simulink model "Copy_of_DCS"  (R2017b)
settings: Solver=FixedStepDiscrete  StartTime=0.0  StopTime=10.0  FixedStep=0.01  RelTol=1e-3  EnableMultiTasking=on
undefined symbols (not defined in the file): ASWTYPE_FALSE, CaDCS_2569BattFctyName_numb, CaDCS_2576SoftVer_numb, CcDCS_2567BattCap_Ah, CcDCS_2568BattVolt_V, CcDCS_2570BattSer_numb, CcDCS_2571BattPrdctDay_D, CcDCS_2571BattPrdctMon_M, CcDCS_2571BattPrdctYr_Y, CcDCS_2572BattChrgCt_numb, CcDCS_2574Resv_numb, CcDCS_2816MaxCellVoltPermit_V, CcDCS_2817MaxCurPermit_A, CcDCS_2818RateEgy_Kwh, CcDCS_2819MaxVoltPermit_V, CcDCS_2820MaxTempPermit_C, CcDCS_3072ChrgVoltReqAdd_V, CcDCS_CMUQnty_numb, CeDCS_2566BattType_enum, CeDCS_2573BattPrpty_enum, CeDCS_3074ChrgMode_enum, CeDCS_FltLevel_enum, DCS_2565Ver_NUMB, DCS_BROAA_NUMB, DCS_CONSTF1_NUMB, DCS_ONE_NUMB, DCS_THOUSAND_NUMB, DCS_ZERO_NUMB, Enum_CTCCtrCtlConnMode, Enum_CTCCtrCtlState, Enum_ISOHVIsoFltLevel, Enum_LDPDCChrgPlugTempState, Enum_SOPChrgPwrState
libraries: AIWAYS_Powertrain_BMS_lib x75
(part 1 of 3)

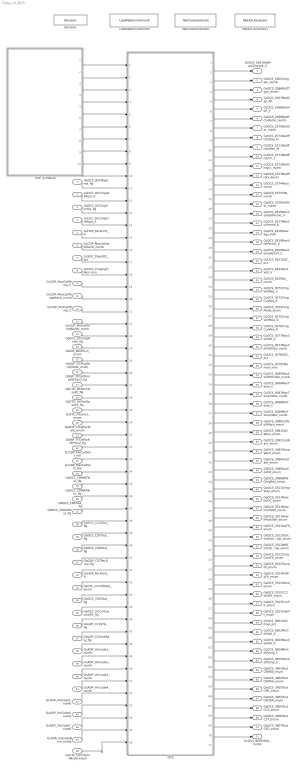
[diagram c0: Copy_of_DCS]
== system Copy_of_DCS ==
  GbDCC_BSTMsgCmd_flg : Inport
  GcDCC_DCChrgVoltRqst_V : Inport  Port=2
  GbDCC_DCChrgVerSta_flg : Inport  Port=3
  GcDCC_DCChrgCrntRqst_A : Inport  Port=4
  GcHDP_PackCrnt_A : Inport  Port=5
  GcCDP_MaxCellVoltNumb_numb : Inport  Port=6
  GcSOC_DispSOC_pct : Inport  Port=7
  GcDCC_ChrgingTiRem_min : Inport  Port=8
  GcCDP_MaxCellTemp_C : Inport  Port=9
  GcCDP_MaxCellTempNumb_numb : Inport  Port=10
  GcCDP_MinCellTemp_C : Inport  Port=11
  GcCDP_MinCellTempNumb_numb : Inport  Port=12
  GbDCC_DCChrgFinish_flg : Inport  Port=13
  GeISO_ResFltLvl_enum : Inport  Port=14
  GeLDP_DCPlugTempState_enum : Inport  Port=15
  GbISP_TFCellTempHiFltLv2_flg : Inport  Port=16
  GbCTD_DCPosCloseFlt_flg : Inport  Port=17
  GbCTD_DCPosOpenFlt_flg : Inport  Port=18
  GeFTC_FltLevel_enum : Inport  Port=19
  GeSOP_ChrgPwrState_enum : Inport  Port=20
  GbISP_TFCellVoltHiFltLv2_flg : Inport  Port=21
  GcCDP_MinCellVolt_mV : Inport  Port=22
  GcCDP_MaxCellVolt_mV : Inport  Port=23
  GbDCC_CRM00Tout_flg : Inport  Port=24
  GbDCC_CRMAATout_flg : Inport  Port=25
  GbDCC_CMLTout_flg : Inport  Port=26
  GbDCC_CROAATout_flg : Inport  Port=27
  GbDCC_CCSTout_flg : Inport  Port=28
  GbDCC_CSTTout_flg : Inport  Port=29
  GbDCC_CSDTout_flg : Inport  Port=30
  GbGDP_CSTRecOnce_flg : Inport  Port=31
  GcHDP_PackVolt_V : Inport  Port=32
  GeCTC_CtrCtlState_enum : Inport  Port=33
  GbDCC_CROTout_flg : Inport  Port=34
  GbDCC_DCCrntUnctrolFlt_flg : Inport  Port=35
  GbLDP_CC2STG_flg : Inport  Port=36
  GbLDP_CC2VoltRaty_flg : Inport  Port=37
  GcADP_VinCode1_numb : Inport  Port=38
  GcADP_VinCode2_numb : Inport  Port=39
  GcADP_VinCode3_numb : Inport  Port=40
  GcADP_VinCode4_numb : Inport  Port=41
  GcADP_VinCode5_numb : Inport  Port=42
  GcADP_VinCode6_numb : Inport  Port=43
  GcADP_VinCode7_numb : Inport  Port=44
  GcADP_VinCodeNum_numb : Inport  Port=45
  GeCTC_CtrCtlConnMode_enum : Inport  Port=46
  DCS : Subsystem
  GDP_Schedule : Stateflow chart  TreatAsAtomicUnit=on
  LoadMptEnvironment : AIWAYS_Powertrain_BMS_lib/Config/LoadMptEnvironment  ProjectName=Comm  SuppierID=NewPlatformUAES
  MptA2LGenerate1 : AIWAYS_Powertrain_BMS_lib/Config/MptA2LGenerate  SystemSampleTime=-1
  MptCodeGenerate1 : AIWAYS_Powertrain_BMS_lib/Config/MptCodeGenerate  SystemSampleTime=-1
  Revision : AIWAYS_Powertrain_BMS_lib/Config/Revision  curVersion='M104C104'  newVersion='M104C104'
  GcDCS_2601AlwMaxChrgVolt_V : Outport
  GcDCS_2565ChrgVer_numb : Outport  Port=2
  GeDCS_2566BattType_enum : Outport  Port=3
  GcDCS_2567BattCap_Ah : Outport  Port=4
  GcDCS_2568BattVolt_V : Outport  Port=5
  GaDCS_2569BattFctyName_numb : Outport  Port=6
  GcDCS_2570BattSer_numb : Outport  Port=7
  GcDCS_2571BattPrdctDay_D : Outport  Port=8
  GcDCS_2571BattPrdctMon_M : Outport  Port=9
  GcDCS_2571BattPrdctYr_Y : Outport  Port=10
  GcDCS_2572BattChrgCt_numb : Outport  Port=11
  GeDCS_2573BattPrpty_enum : Outport  Port=12
  GcDCS_2574Resv_numb : Outport  Port=13
  GaDCS_2575VIN_numb : Outport  Port=14
  GaDCS_2576SoftVer_numb : Outport  Port=15
  GcDCS_2816MaxCellVoltPermit_V : Outport  Port=16
  GcDCS_2817MaxCurPermit_A : Outport  Port=17
  GcDCS_2818RateEgy_Kwh : Outport  Port=18
  GcDCS_2819MaxVoltPermit_V : Outport  Port=19
  GcDCS_2820MaxTempPermit_C : Outport  Port=20
  GcDCS_2821SOC_pct : Outport  Port=21
  GcDCS_2822PackVolt_V : Outport  Port=22
  GcDCS_2829Da_numb : Outport  Port=23
  GcDCS_3072ChrgVoltReq_V : Outport  Port=24
  GcDCS_3073ChrgCurReq_A : Outport  Port=25
  GeDCS_3074ChrgMode_enum : Outport  Port=26
  GcDCS_3075ChrgVoltMea_V : Outport  Port=27
  GcDCS_3076ChrgCurMea_A : Outport  Port=28
  GcDCS_3077MaxCellVolt_V : Outport  Port=29
  GcDCS_3077MaxCellVoltGrp_numb : Outport  Port=30
  GcDCS_3078SOC_pct : Outport  Port=31
  GcDCS_3079TiRemain_min : Outport  Port=32
  GcDCS_3085MaxCellVoltIndex_numb : Outport  Port=33
  GcDCS_3086MaxTemp_C : Outport  Port=34
  GcDCS_3087MaxTempIndex_numb : Outport  Port=35
  GcDCS_3088MinTemp_C : Outport  Port=36
  GcDCS_3089MinTempIndex_numb : Outport  Port=37
  GeDCS_3090CellVoltWarn_enum : Outport  Port=38
  GeDCS_3091SOCWarn_enum : Outport  Port=39
  GeDCS_3092CurWarn_enum : Outport  Port=40
  GeDCS_3093TempWarn_enum : Outport  Port=41
  GeDCS_3094IsoState_enum : Outport  Port=42
  GeDCS_3095OutContSt_enum : Outport  Port=43
  GeDCS_3096BMSChrgRdy_enum : Outport  Port=44
  GeDCS_3511ChrgrStop_enum : Outport  Port=45
  GeDCS_3511ReachSOC_enum : Outport  Port=46
  GeDCS_3511ReachCellVolt_enum : Outport  Port=47
  GeDCS_3511ReachPackVolt_enum : Outport  Port=48
  GeDCS_3512IsoFlt_enum : Outport  Port=49
  GeDCS_3512OutContOverTemp_enum : Outport  Port=50
  GeDCS_3512BMSCompOverTemp_enum : Outport  Port=51
  GeDCS_3512ChrgContFlt_enum : Outport  Port=52
  GeDCS_3512TempFlt_enum : Outport  Port=53
  GeDCS_3512HVRlyFlt_enum : Outport  Port=54
  GeDCS_3512Other_enum : Outport  Port=55
  GeDCS_3512CC2VoltFlt_enum : Outport  Port=56
  GeDCS_3513CurrFlt_enum : Outport  Port=57
  GeDCS_3513VoltFlt_enum : Outport  Port=58
  GcDCS_3601SOCFinal_pct : Outport  Port=59
  GcDCS_3602MinCellVolt_V : Outport  Port=60
  GcDCS_3603MaxCellVolt_V : Outport  Port=61
  GcDCS_3604MinCellTemp_C : Outport  Port=62
  GcDCS_3605MaxCellTemp_C : Outport  Port=63
  GeDCS_3901ToutCRM00_enum : Outport  Port=64
  GeDCS_3902ToutCRMAA_enum : Outport  Port=65
  GeDCS_3903ToutCML_enum : Outport  Port=66
  GeDCS_3904ToutCROAA_enum : Outport  Port=67
  GeDCS_3905ToutCCS_enum : Outport  Port=68
  GeDCS_3906ToutCST_enum : Outport  Port=69
  GeDCS_3907ToutCSD_enum : Outport  Port=70
  GcDCS_BEMOther_numb : Outport  Port=71
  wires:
  DCS/1(GcDCS_2601AlwMaxChrgVolt_V) -> GcDCS_2601AlwMaxChrgVolt_V/1
  DCS/2(GcDCS_2565ChrgVer_numb) -> GcDCS_2565ChrgVer_numb/1
  DCS/3(GeDCS_2566BattType_enum) -> GeDCS_2566BattType_enum/1
  DCS/4(GcDCS_2567BattCap_Ah) -> GcDCS_2567BattCap_Ah/1
  DCS/5(GcDCS_2568BattVolt_V) -> GcDCS_2568BattVolt_V/1
  DCS/6(GaDCS_2569BattFctyName_numb) -> GaDCS_2569BattFctyName_numb/1
  DCS/7(GcDCS_2570BattSer_numb) -> GcDCS_2570BattSer_numb/1
  DCS/8(GcDCS_2571BattPrdctDay_D) -> GcDCS_2571BattPrdctDay_D/1
  DCS/9(GcDCS_2571BattPrdctMon_M) -> GcDCS_2571BattPrdctMon_M/1
  DCS/10(GcDCS_2571BattPrdctYr_Y) -> GcDCS_2571BattPrdctYr_Y/1
  DCS/11(GcDCS_2572BattChrgCt_numb) -> GcDCS_2572BattChrgCt_numb/1
  DCS/12(GeDCS_2573BattPrpty_enum) -> GeDCS_2573BattPrpty_enum/1
  DCS/13(GcDCS_2574Resv_numb) -> GcDCS_2574Resv_numb/1
  DCS/14(GaDCS_2575VIN_numb) -> GaDCS_2575VIN_numb/1
  DCS/15(GaDCS_2576SoftVer_numb) -> GaDCS_2576SoftVer_numb/1
  DCS/16(GcDCS_2816MaxCellVoltPermit_V) -> GcDCS_2816MaxCellVoltPermit_V/1
  DCS/17(GcDCS_2817MaxCurPermit_A) -> GcDCS_2817MaxCurPermit_A/1
  DCS/18(GcDCS_2818RateEgy_Kwh) -> GcDCS_2818RateEgy_Kwh/1
  DCS/19(GcDCS_2819MaxVoltPermit_V) -> GcDCS_2819MaxVoltPermit_V/1
  DCS/20(GcDCS_2820MaxTempPermit_C) -> GcDCS_2820MaxTempPermit_C/1
  DCS/21(GcDCS_2821SOC_pct) -> GcDCS_2821SOC_pct/1
  DCS/22(GcDCS_2822PackVolt_V) -> GcDCS_2822PackVolt_V/1
  DCS/23(GcDCS_2829Da_numb) -> GcDCS_2829Da_numb/1
  DCS/24(GcDCS_3072ChrgVoltReq_V) -> GcDCS_3072ChrgVoltReq_V/1
  DCS/25(GcDCS_3073ChrgCurReq_A) -> GcDCS_3073ChrgCurReq_A/1
  DCS/26(GeDCS_3074ChrgMode_enum) -> GeDCS_3074ChrgMode_enum/1
  DCS/27(GcDCS_3075ChrgVoltMea_V) -> GcDCS_3075ChrgVoltMea_V/1
  DCS/28(GcDCS_3076ChrgCurMea_A) -> GcDCS_3076ChrgCurMea_A/1
  DCS/29(GcDCS_3077MaxCellVolt_V) -> GcDCS_3077MaxCellVolt_V/1
  DCS/30(GcDCS_3077MaxCellVoltGrp_numb) -> GcDCS_3077MaxCellVoltGrp_numb/1
  DCS/31(GcDCS_3078SOC_pct) -> GcDCS_3078SOC_pct/1
  DCS/32(GcDCS_3079TiRemain_min) -> GcDCS_3079TiRemain_min/1
  DCS/33(GcDCS_3085MaxCellVoltIndex_numb) -> GcDCS_3085MaxCellVoltIndex_numb/1
  DCS/34(GcDCS_3086MaxTemp_C) -> GcDCS_3086MaxTemp_C/1
  DCS/35(GcDCS_3087MaxTempIndex_numb) -> GcDCS_3087MaxTempIndex_numb/1
  DCS/36(GcDCS_3088MinTemp_C) -> GcDCS_3088MinTemp_C/1
  DCS/37(GcDCS_3089MinTempIndex_numb) -> GcDCS_3089MinTempIndex_numb/1
  DCS/38(GeDCS_3090CellVoltWarn_enum) -> GeDCS_3090CellVoltWarn_enum/1
  DCS/39(GeDCS_3091SOCWarn_enum) -> GeDCS_3091SOCWarn_enum/1
  DCS/40(GeDCS_3092CurWarn_enum) -> GeDCS_3092CurWarn_enum/1
  DCS/41(GeDCS_3093TempWarn_enum) -> GeDCS_3093TempWarn_enum/1
  DCS/42(GeDCS_3094IsoState_enum) -> GeDCS_3094IsoState_enum/1
  DCS/43(GeDCS_3095OutContSt_enum) -> GeDCS_3095OutContSt_enum/1
  DCS/44(GeDCS_3096BMSChrgRdy_enum) -> GeDCS_3096BMSChrgRdy_enum/1
  DCS/45(GeDCS_3511ChrgrStop_enum) -> GeDCS_3511ChrgrStop_enum/1
  DCS/46(GeDCS_3511ReachSOC_enum) -> GeDCS_3511ReachSOC_enum/1
  DCS/47(GeDCS_3511ReachCellVolt_enum) -> GeDCS_3511ReachCellVolt_enum/1
  DCS/48(GeDCS_3511ReachPackVolt_enum) -> GeDCS_3511ReachPackVolt_enum/1
  DCS/49(GeDCS_3512IsoFlt_enum) -> GeDCS_3512IsoFlt_enum/1
  DCS/50(GeDCS_3512OutContOverTemp_enum) -> GeDCS_3512OutContOverTemp_enum/1
  DCS/51(GeDCS_3512BMSCompOverTemp_enum) -> GeDCS_3512BMSCompOverTemp_enum/1
  DCS/52(GeDCS_3512ChrgContFlt_enum) -> GeDCS_3512ChrgContFlt_enum/1
  DCS/53(GeDCS_3512TempFlt_enum) -> GeDCS_3512TempFlt_enum/1
  DCS/54(GeDCS_3512HVRlyFlt_enum) -> GeDCS_3512HVRlyFlt_enum/1
  DCS/55(GeDCS_3512Other_enum) -> GeDCS_3512Other_enum/1
  DCS/56(GeDCS_3512CC2VoltFlt_enum) -> GeDCS_3512CC2VoltFlt_enum/1
  DCS/57(GeDCS_3513CurrFlt_enum) -> GeDCS_3513CurrFlt_enum/1
  DCS/58(GeDCS_3513VoltFlt_enum) -> GeDCS_3513VoltFlt_enum/1
  DCS/59(GcDCS_3601SOCFinal_pct) -> GcDCS_3601SOCFinal_pct/1
  DCS/60(GcDCS_3602MinCellVolt_V) -> GcDCS_3602MinCellVolt_V/1
  DCS/61(GcDCS_3603MaxCellVolt_V) -> GcDCS_3603MaxCellVolt_V/1
  DCS/62(GcDCS_3604MinCellTemp_C) -> GcDCS_3604MinCellTemp_C/1
  DCS/63(GcDCS_3605MaxCellTemp_C) -> GcDCS_3605MaxCellTemp_C/1
  DCS/64(GeDCS_3901ToutCRM00_enum) -> GeDCS_3901ToutCRM00_enum/1
  DCS/65(GeDCS_3902ToutCRMAA_enum) -> GeDCS_3902ToutCRMAA_enum/1
  DCS/66(GeDCS_3903ToutCML_enum) -> GeDCS_3903ToutCML_enum/1
  DCS/67(GeDCS_3904ToutCROAA_enum) -> GeDCS_3904ToutCROAA_enum/1
  DCS/68(GeDCS_3905ToutCCS_enum) -> GeDCS_3905ToutCCS_enum/1
  DCS/69(GeDCS_3906ToutCST_enum) -> GeDCS_3906ToutCST_enum/1
  DCS/70(GeDCS_3907ToutCSD_enum) -> GeDCS_3907ToutCSD_enum/1
  DCS/71(GcDCS_BEMOther_numb) -> GcDCS_BEMOther_numb/1
  GDP_Schedule/1(DCS_BST_10ms()) -> DCS/1(DCS_BST_10ms)
  GDP_Schedule/2(DCS_BCL_50ms()) -> DCS/2(DCS_BCL_50ms)
  GDP_Schedule/3(DCS_BHM_250ms()) -> DCS/3(DCS_BHM_250ms)
  GDP_Schedule/4(DCS_BRM_250ms()) -> DCS/4(DCS_BRM_250ms)
  GDP_Schedule/5(DCS_BRO_250ms()) -> DCS/5(DCS_BRO_250ms)
  GDP_Schedule/6(DCS_BCS_250ms()) -> DCS/6(DCS_BCS_250ms)
  GDP_Schedule/7(DCS_BSM_250ms()) -> DCS/7(DCS_BSM_250ms)
  GDP_Schedule/8(DCS_BSD_250ms()) -> DCS/8(DCS_BSD_250ms)
  GDP_Schedule/9(DCS_BEM_250ms()) -> DCS/9(DCS_BEM_250ms)
  GDP_Schedule/10(DCS_BCP_500ms()) -> DCS/10(DCS_BCP_500ms)
  GbDCC_BSTMsgCmd_flg/1 -> DCS/11(GbDCC_BSTMsgCmd_flg)
  GcDCC_DCChrgVoltRqst_V/1 -> DCS/12(GcDCC_DCChrgVoltRqst_V)
  GbDCC_DCChrgVerSta_flg/1 -> DCS/13(GbDCC_DCChrgVerSta_flg)
  GcDCC_DCChrgCrntRqst_A/1 -> DCS/14(GcDCC_DCChrgCrntRqst_A)
  GcHDP_PackCrnt_A/1 -> DCS/15(GcHDP_PackCrnt_A)
  GcCDP_MaxCellVoltNumb_numb/1 -> DCS/16(GcCDP_MaxCellVoltNumb_numb)
  GcSOC_DispSOC_pct/1 -> DCS/17(GcSOC_DispSOC_pct)
  GcDCC_ChrgingTiRem_min/1 -> DCS/18(GcDCC_ChrgingTiRem_min)
  GcCDP_MaxCellTemp_C/1 -> DCS/19(GcCDP_MaxCellTemp_C)
  GcCDP_MaxCellTempNumb_numb/1 -> DCS/20(GcCDP_MaxCellTempNumb_numb)
  GcCDP_MinCellTemp_C/1 -> DCS/21(GcCDP_MinCellTemp_C)
  GcCDP_MinCellTempNumb_numb/1 -> DCS/22(GcCDP_MinCellTempNumb_numb)
  GbDCC_DCChrgFinish_flg/1 -> DCS/23(GbDCC_DCChrgFinish_flg)
  GeISO_ResFltLvl_enum/1 -> DCS/24(GeISO_ResFltLvl_enum)
  GeLDP_DCPlugTempState_enum/1 -> DCS/25(GeLDP_DCPlugTempState_enum)
  GbISP_TFCellTempHiFltLv2_flg/1 -> DCS/26(GbISP_TFCellTempHiFltLv2_flg)
  GbCTD_DCPosCloseFlt_flg/1 -> DCS/27(GbCTD_DCPosCloseFlt_flg)
  GbCTD_DCPosOpenFlt_flg/1 -> DCS/28(GbCTD_DCPosOpenFlt_flg)
  GeFTC_FltLevel_enum/1 -> DCS/29(GeFTC_FltLevel_enum)
  GeSOP_ChrgPwrState_enum/1 -> DCS/30(GeSOP_ChrgPwrState_enum)
  GbISP_TFCellVoltHiFltLv2_flg/1 -> DCS/31(GbISP_TFCellVoltHiFltLv2_flg)
  GcCDP_MinCellVolt_mV/1 -> DCS/32(GcCDP_MinCellVolt_mV)
  GcCDP_MaxCellVolt_mV/1 -> DCS/33(GcCDP_MaxCellVolt_mV)
  GbDCC_CRM00Tout_flg/1 -> DCS/34(GbDCC_CRM00Tout_flg)
  GbDCC_CRMAATout_flg/1 -> DCS/35(GbDCC_CRMAATout_flg)
  GbDCC_CMLTout_flg/1 -> DCS/36(GbDCC_CMLTout_flg)
  GbDCC_CROAATout_flg/1 -> DCS/37(GbDCC_CROAATout_flg)
  GbDCC_CCSTout_flg/1 -> DCS/38(GbDCC_CCSTout_flg)
  GbDCC_CSTTout_flg/1 -> DCS/39(GbDCC_CSTTout_flg)
  GbDCC_CSDTout_flg/1 -> DCS/40(GbDCC_CSDTout_flg)
  GbGDP_CSTRecOnce_flg/1 -> DCS/41(GbGDP_CSTRecOnce_flg)
  GcHDP_PackVolt_V/1 -> DCS/42(GcHDP_PackVolt_V)
  GeCTC_CtrCtlState_enum/1 -> DCS/43(GeCTC_CtrCtlState_enum)
  GbDCC_CROTout_flg/1 -> DCS/44(GbDCC_CROTout_flg)
  GbDCC_DCCrntUnctrolFlt_flg/1 -> DCS/45(GbDCC_DCCrntUnctrolFlt_flg)
  GbLDP_CC2STG_flg/1 -> DCS/46(GbLDP_CC2STG_flg)
  GbLDP_CC2VoltRaty_flg/1 -> DCS/47(GbLDP_CC2VoltRaty_flg)
  GcADP_VinCode1_numb/1 -> DCS/48(GcADP_VinCode1_numb)
  GcADP_VinCode2_numb/1 -> DCS/49(GcADP_VinCode2_numb)
  GcADP_VinCode3_numb/1 -> DCS/50(GcADP_VinCode3_numb)
  GcADP_VinCode4_numb/1 -> DCS/51(GcADP_VinCode4_numb)
  GcADP_VinCode5_numb/1 -> DCS/52(GcADP_VinCode5_numb)
  GcADP_VinCode6_numb/1 -> DCS/53(GcADP_VinCode6_numb)
  GcADP_VinCode7_numb/1 -> DCS/54(GcADP_VinCode7_numb)
  GcADP_VinCodeNum_numb/1 -> DCS/55(GcADP_VinCodeNum_numb)
  GeCTC_CtrCtlConnMode_enum/1 -> DCS/56(GeCTC_CtrCtlConnMode_enum)

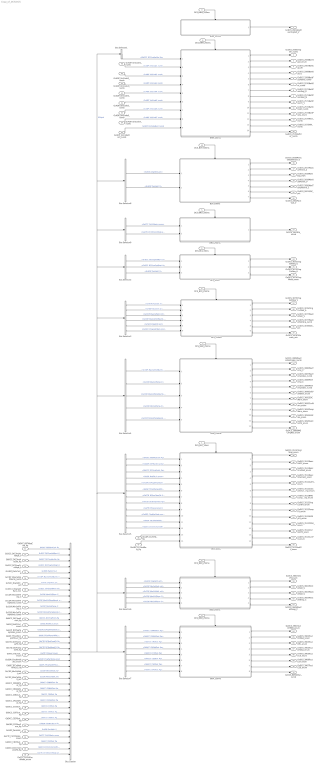
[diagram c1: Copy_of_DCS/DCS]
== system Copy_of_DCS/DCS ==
  DCS_BST_10ms : Inport
  DCS_BCL_50ms : Inport  Port=2
  DCS_BHM_250ms : Inport  Port=3
  DCS_BRM_250ms : Inport  Port=4
  DCS_BRO_250ms : Inport  Port=5
  DCS_BCS_250ms : Inport  Port=6
  DCS_BSM_250ms : Inport  Port=7
  DCS_BSD_250ms : Inport  Port=8
  DCS_BEM_250ms : Inport  Port=9
  DCS_BCP_500ms : Inport  Port=10
  GbDCC_BSTMsgCmd_flg : Inport  Port=11
  GcDCC_DCChrgVoltRqst_V : Inport  Port=12
  GbDCC_DCChrgVerSta_flg : Inport  Port=13
  GcDCC_DCChrgCrntRqst_A : Inport  Port=14
  GcHDP_PackCrnt_A : Inport  Port=15
  GcCDP_MaxCellVoltNumb_numb : Inport  Port=16
  GcSOC_DispSOC_pct : Inport  Port=17
  GcDCC_ChrgingTiRem_min : Inport  Port=18
  GcCDP_MaxCellTemp_C : Inport  Port=19
  GcCDP_MaxCellTempNumb_numb : Inport  Port=20
  GcCDP_MinCellTemp_C : Inport  Port=21
  GcCDP_MinCellTempNumb_numb : Inport  Port=22
  GbDCC_DCChrgFinish_flg : Inport  Port=23
  GeISO_ResFltLvl_enum : Inport  Port=24
  GeLDP_DCPlugTempState_enum : Inport  Port=25
  GbISP_TFCellTempHiFltLv2_flg : Inport  Port=26
  GbCTD_DCPosCloseFlt_flg : Inport  Port=27
  GbCTD_DCPosOpenFlt_flg : Inport  Port=28
  GeFTC_FltLevel_enum : Inport  Port=29
  GeSOP_ChrgPwrState_enum : Inport  Port=30
  GbISP_TFCellVoltHiFltLv2_flg : Inport  Port=31
  GcCDP_MinCellVolt_mV : Inport  Port=32
  GcCDP_MaxCellVolt_mV : Inport  Port=33
  GbDCC_CRM00Tout_flg : Inport  Port=34
  GbDCC_CRMAATout_flg : Inport  Port=35
  GbDCC_CMLTout_flg : Inport  Port=36
  GbDCC_CROAATout_flg : Inport  Port=37
  GbDCC_CCSTout_flg : Inport  Port=38
  GbDCC_CSTTout_flg : Inport  Port=39
  GbDCC_CSDTout_flg : Inport  Port=40
  GbGDP_CSTRecOnce_flg : Inport  Port=41
  GcHDP_PackVolt_V : Inport  Port=42
  GeCTC_CtrCtlState_enum : Inport  Port=43
  GbDCC_CROTout_flg : Inport  Port=44
  GbDCC_DCCrntUnctrolFlt_flg : Inport  Port=45
  GbLDP_CC2STG_flg : Inport  Port=46
  GbLDP_CC2VoltRaty_flg : Inport  Port=47
  GcADP_VinCode1_numb : Inport  Port=48
  GcADP_VinCode2_numb : Inport  Port=49
  GcADP_VinCode3_numb : Inport  Port=50
  GcADP_VinCode4_numb : Inport  Port=51
  GcADP_VinCode5_numb : Inport  Port=52
  GcADP_VinCode6_numb : Inport  Port=53
  GcADP_VinCode7_numb : Inport  Port=54
  GcADP_VinCodeNum_numb : Inport  Port=55
  GeCTC_CtrCtlConnMode_enum : Inport  Port=56
  BCL_50ms : Subsystem
  BCP_500ms : Subsystem
  BCS_250ms : Subsystem
  BEM_250ms : Subsystem
  BHM_250ms : Subsystem
  BRM_250ms : Subsystem
  BRO_250ms : Subsystem
  BSD_250ms : Subsystem
  BSM_250ms : Subsystem
  BST_10ms : Subsystem
  Bus Creator : BusCreator  Inputs=36
  Bus Selector1 : BusSelector  OutputSignals=GbDCC_DCChrgVerSta_flg
  Bus Selector2 : BusSelector  OutputSignals=GcDCC_DCChrgVoltRqst_V,GcDCC_DCChrgCrntRqst_A,GcHDP_PackVolt_V
  Bus Selector3 : BusSelector  OutputSignals=GcHDP_PackVolt_V,GcHDP_PackCrnt_A,GcCDP_MaxCellVolt_mV,GcCDP_MaxCellVoltNumb_numb,GcSOC_DispSOC_pct,GcDCC_ChrgingTiRem_min
  Bus Selector4 : BusSelector  OutputSignals=GcCDP_MaxCellVoltNumb_numb,GcCDP_MaxCellTemp_C,GcCDP_MaxCellTempNumb_numb,GcCDP_MinCellTemp_C,GcCDP_MinCellTempNumb_numb
  Bus Selector5 : BusSelector  OutputSignals=GbDCC_BSTMsgCmd_flg,GbGDP_CSTRecOnce_flg,GbDCC_DCChrgFinish_flg,GeISO_ResFltLvl_enum,GeLDP_DCPlugTempState_enum,GbISP_TFCellTempHiFltLv2_flg,GbCTD_DCPosCloseFlt_flg,GbCTD_DCPosOpenFlt_flg,GeFTC_FltLevel_enum,GeSOP_ChrgPwrState_enum,GbISP_TFCellVoltHiFltLv2_flg,GbDCC_DCCrntUnctrolFlt_flg
  Bus Selector6 : BusSelector  OutputSignals=GcSOC_DispSOC_pct,GcCDP_MinCellVolt_mV,GcCDP_MaxCellVolt_mV,GcCDP_MaxCellTemp_C,GcCDP_MinCellTemp_C
  Bus Selector7 : BusSelector  OutputSignals=GbDCC_CRM00Tout_flg,GbDCC_CRMAATout_flg,GbDCC_CMLTout_flg,GbDCC_CROAATout_flg,GbDCC_CCSTout_flg,GbDCC_CSTTout_flg,GbDCC_CSDTout_flg,GbDCC_CROTout_flg
  Bus Selector8 : BusSelector  OutputSignals=GcSOC_DispSOC_pct,GcHDP_PackVolt_V
  Bus Selector9 : BusSelector  OutputSignals=GeCTC_CtrCtlState_enum,GeCTC_CtrCtlConnMode_enum
  GcDCS_2601AlwMaxChrgVolt_V : Outport
  GcDCS_2565ChrgVer_numb : Outport  Port=2
  GeDCS_2566BattType_enum : Outport  Port=3
  GcDCS_2567BattCap_Ah : Outport  Port=4
  GcDCS_2568BattVolt_V : Outport  Port=5
  GaDCS_2569BattFctyName_numb : Outport  Port=6
  GcDCS_2570BattSer_numb : Outport  Port=7
  GcDCS_2571BattPrdctDay_D : Outport  Port=8
  GcDCS_2571BattPrdctMon_M : Outport  Port=9
  GcDCS_2571BattPrdctYr_Y : Outport  Port=10
  GcDCS_2572BattChrgCt_numb : Outport  Port=11
  GeDCS_2573BattPrpty_enum : Outport  Port=12
  GcDCS_2574Resv_numb : Outport  Port=13
  GaDCS_2575VIN_numb : Outport  Port=14
  GaDCS_2576SoftVer_numb : Outport  Port=15
  GcDCS_2816MaxCellVoltPermit_V : Outport  Port=16
  GcDCS_2817MaxCurPermit_A : Outport  Port=17
  GcDCS_2818RateEgy_Kwh : Outport  Port=18
  GcDCS_2819MaxVoltPermit_V : Outport  Port=19
  GcDCS_2820MaxTempPermit_C : Outport  Port=20
  GcDCS_2821SOC_pct : Outport  Port=21
  GcDCS_2822PackVolt_V : Outport  Port=22
  GcDCS_2829Da_numb : Outport  Port=23
  GcDCS_3072ChrgVoltReq_V : Outport  Port=24
  GcDCS_3073ChrgCurReq_A : Outport  Port=25
  GeDCS_3074ChrgMode_enum : Outport  Port=26
  GcDCS_3075ChrgVoltMea_V : Outport  Port=27
  GcDCS_3076ChrgCurMea_A : Outport  Port=28
  GcDCS_3077MaxCellVolt_V : Outport  Port=29
  GcDCS_3077MaxCellVoltGrp_numb : Outport  Port=30
  GcDCS_3078SOC_pct : Outport  Port=31
  GcDCS_3079TiRemain_min : Outport  Port=32
  GcDCS_3085MaxCellVoltIndex_numb : Outport  Port=33
  GcDCS_3086MaxTemp_C : Outport  Port=34
  GcDCS_3087MaxTempIndex_numb : Outport  Port=35
  GcDCS_3088MinTemp_C : Outport  Port=36
  GcDCS_3089MinTempIndex_numb : Outport  Port=37
  GeDCS_3090CellVoltWarn_enum : Outport  Port=38
  GeDCS_3091SOCWarn_enum : Outport  Port=39
  GeDCS_3092CurWarn_enum : Outport  Port=40
  GeDCS_3093TempWarn_enum : Outport  Port=41
  GeDCS_3094IsoState_enum : Outport  Port=42
  GeDCS_3095OutContSt_enum : Outport  Port=43
  GeDCS_3096BMSChrgRdy_enum : Outport  Port=44
  GeDCS_3511ChrgrStop_enum : Outport  Port=45
  GeDCS_3511ReachSOC_enum : Outport  Port=46
  GeDCS_3511ReachCellVolt_enum : Outport  Port=47
  GeDCS_3511ReachPackVolt_enum : Outport  Port=48
  GeDCS_3512IsoFlt_enum : Outport  Port=49
  GeDCS_3512OutContOverTemp_enum : Outport  Port=50
  GeDCS_3512BMSCompOverTemp_enum : Outport  Port=51
  GeDCS_3512ChrgContFlt_enum : Outport  Port=52
  GeDCS_3512TempFlt_enum : Outport  Port=53
  GeDCS_3512HVRlyFlt_enum : Outport  Port=54
  GeDCS_3512Other_enum : Outport  Port=55
  GeDCS_3512CC2VoltFlt_enum : Outport  Port=56
  GeDCS_3513CurrFlt_enum : Outport  Port=57
  GeDCS_3513VoltFlt_enum : Outport  Port=58
  GcDCS_3601SOCFinal_pct : Outport  Port=59
  GcDCS_3602MinCellVolt_V : Outport  Port=60
  GcDCS_3603MaxCellVolt_V : Outport  Port=61
  GcDCS_3604MinCellTemp_C : Outport  Port=62
  GcDCS_3605MaxCellTemp_C : Outport  Port=63
  GeDCS_3901ToutCRM00_enum : Outport  Port=64
  GeDCS_3902ToutCRMAA_enum : Outport  Port=65
  GeDCS_3903ToutCML_enum : Outport  Port=66
  GeDCS_3904ToutCROAA_enum : Outport  Port=67
  GeDCS_3905ToutCCS_enum : Outport  Port=68
  GeDCS_3906ToutCST_enum : Outport  Port=69
  GeDCS_3907ToutCSD_enum : Outport  Port=70
  GcDCS_BEMOther_numb : Outport  Port=71
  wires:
  BSD_250ms/4(GcDCS_3604MinCellTemp_C) -> GcDCS_3604MinCellTemp_C/1
  BSD_250ms/3(GcDCS_3603MaxCellVolt_V) -> GcDCS_3603MaxCellVolt_V/1
  BSD_250ms/2(GcDCS_3602MinCellVolt_V) -> GcDCS_3602MinCellVolt_V/1
  BSD_250ms/5(GcDCS_3605MaxCellTemp_C) -> GcDCS_3605MaxCellTemp_C/1
  BSD_250ms/1(GcDCS_3601SOCFinal_pct) -> GcDCS_3601SOCFinal_pct/1
  GcDCC_DCChrgVoltRqst_V/1 -> Bus Creator/2  "GcDCC_DCChrgVoltRqst_V"
  GbDCC_DCChrgVerSta_flg/1 -> Bus Creator/3  "GbDCC_DCChrgVerSta_flg"
  GcDCC_DCChrgCrntRqst_A/1 -> Bus Creator/4  "GcDCC_DCChrgCrntRqst_A"
  Bus Selector1/1 -> BRM_250ms/1(GbDCC_DCChrgVerSta_flg)  "<GbDCC_DCChrgVerSta_flg>"
  Bus Selector4/5 -> BSM_250ms/5(GcCDP_MinCellTempNumb_numb)  "<GcCDP_MinCellTempNumb_numb>"
  Bus Selector4/2 -> BSM_250ms/2(GcCDP_MaxCellTemp_C)  "<GcCDP_MaxCellTemp_C>"
  Bus Selector4/4 -> BSM_250ms/4(GcCDP_MinCellTemp_C)  "<GcCDP_MinCellTemp_C>"
  Bus Selector3/1 -> BCS_250ms/1(GcHDP_PackVolt_V)  "<GcHDP_PackVolt_V>"
  Bus Selector4/1 -> BSM_250ms/1(GcCDP_MaxCellVoltNumb_numb)  "<GcCDP_MaxCellVoltNumb_numb>"
  Bus Selector3/2 -> BCS_250ms/2(GcHDP_PackCrnt_A)  "<GcHDP_PackCrnt_A>"
  Bus Selector3/3 -> BCS_250ms/3(GcCDP_MaxCellVolt_mV)  "<GcCDP_MaxCellVolt_mV>"
  Bus Selector2/1 -> BCL_50ms/1(GcDCC_DCChrgVoltRqst_V)  "<GcDCC_DCChrgVoltRqst_V>"
  Bus Selector3/6 -> BCS_250ms/6(GcDCC_ChrgingTiRem_min)  "<GcDCC_ChrgingTiRem_min>"
  Bus Selector3/5 -> BCS_250ms/5(GcSOC_DispSOC_pct)  "<GcSOC_DispSOC_pct>"
  Bus Selector2/2 -> BCL_50ms/2(GcDCC_DCChrgCrntRqst_A)  "<GcDCC_DCChrgCrntRqst_A>"
  Bus Selector3/4 -> BCS_250ms/4(GcCDP_MaxCellVoltNumb_numb)  "<GcCDP_MaxCellVoltNumb_numb>"
  Bus Selector4/3 -> BSM_250ms/3(GcCDP_MaxCellTempNumb_numb)  "<GcCDP_MaxCellTempNumb_numb>"
  Bus Selector5/5 -> BST_10ms/5(GeLDP_DCPlugTempState_enum)  "<GeLDP_DCPlugTempState_enum>"
  BRM_250ms/10(GcDCS_2572BattChrgCt_numb) -> GcDCS_2572BattChrgCt_numb/1
  BRM_250ms/3(GcDCS_2567BattCap_Ah) -> GcDCS_2567BattCap_Ah/1
  BRM_250ms/11(GeDCS_2573BattPrpty_enum) -> GeDCS_2573BattPrpty_enum/1
  Bus Selector7/5 -> BEM_250ms/5(GbDCC_CCSTout_flg)  "<GbDCC_CCSTout_flg>"
  BRM_250ms/9(GcDCS_2571BattPrdctYr_Y) -> GcDCS_2571BattPrdctYr_Y/1
  Bus Selector7/3 -> BEM_250ms/3(GbDCC_CMLTout_flg)  "<GbDCC_CMLTout_flg>"
  Bus Selector7/2 -> BEM_250ms/2(GbDCC_CRMAATout_flg)  "<GbDCC_CRMAATout_flg>"
  Bus Selector6/4 -> BSD_250ms/4(GcCDP_MaxCellTemp_C)  "<GcCDP_MaxCellTemp_C>"
  BRM_250ms/4(GcDCS_2568BattVolt_V) -> GcDCS_2568BattVolt_V/1
  BRM_250ms/6(GcDCS_2570BattSer_numb) -> GcDCS_2570BattSer_numb/1
  BRM_250ms/14(GaDCS_2576SoftVer_numb) -> GaDCS_2576SoftVer_numb/1
  BRM_250ms/1(GcDCS_2565ChrgVer_numb) -> GcDCS_2565ChrgVer_numb/1
  BHM_250ms/1(GcDCS_2601AlwMaxChrgVolt_V) -> GcDCS_2601AlwMaxChrgVolt_V/1
  Bus Selector6/3 -> BSD_250ms/3(GcCDP_MaxCellVolt_mV)  "<GcCDP_MaxCellVolt_mV>"
  BRM_250ms/13(GaDCS_2575VIN_numb) -> GaDCS_2575VIN_numb/1
  Bus Selector7/6 -> BEM_250ms/6(GbDCC_CSTTout_flg)  "<GbDCC_CSTTout_flg>"
  Bus Selector5/9 -> BST_10ms/9(GeFTC_FltLevel_enum)  "<GeFTC_FltLevel_enum>"
  Bus Selector5/6 -> BST_10ms/6(GbISP_TFCellTempHiFltLv2_flg)  "<GbISP_TFCellTempHiFltLv2_flg>"
  Bus Selector6/2 -> BSD_250ms/2(GcCDP_MinCellVolt_mV)  "<GcCDP_MinCellVolt_mV>"
  Bus Selector6/5 -> BSD_250ms/5(GcCDP_MinCellTemp_C)  "<GcCDP_MinCellTemp_C>"
  BRM_250ms/8(GcDCS_2571BattPrdctMon_M) -> GcDCS_2571BattPrdctMon_M/1
  BRM_250ms/5(GaDCS_2569BattFctyName_numb) -> GaDCS_2569BattFctyName_numb/1
  BRM_250ms/2(GeDCS_2566BattType_enum) -> GeDCS_2566BattType_enum/1
  Bus Selector7/1 -> BEM_250ms/1(GbDCC_CRM00Tout_flg)  "<GbDCC_CRM00Tout_flg>"
  Bus Selector7/7 -> BEM_250ms/7(GbDCC_CSDTout_flg)  "<GbDCC_CSDTout_flg>"
  Bus Selector5/10 -> BST_10ms/10(GeSOP_ChrgPwrState_enum)  "<GeSOP_ChrgPwrState_enum>"
  BRM_250ms/7(GcDCS_2571BattPrdctDay_D) -> GcDCS_2571BattPrdctDay_D/1
  Bus Selector7/4 -> BEM_250ms/4(GbDCC_CROAATout_flg)  "<GbDCC_CROAATout_flg>"
  Bus Selector5/8 -> BST_10ms/8(GbCTD_DCPosOpenFlt_flg)  "<GbCTD_DCPosOpenFlt_flg>"
  Bus Selector5/2 -> BST_10ms/2(GbGDP_CSTRecOnce_flg)  "<GbGDP_CSTRecOnce_flg>"
  Bus Selector5/4 -> BST_10ms/4(GeISO_ResFltLvl_enum)  "<GeISO_ResFltLvl_enum>"
  BRM_250ms/12(GcDCS_2574Resv_numb) -> GcDCS_2574Resv_numb/1
  Bus Selector5/7 -> BST_10ms/7(GbCTD_DCPosCloseFlt_flg)  "<GbCTD_DCPosCloseFlt_flg>"
  Bus Selector5/3 -> BST_10ms/3(GbDCC_DCChrgFinish_flg)  "<GbDCC_DCChrgFinish_flg>"
  Bus Selector5/11 -> BST_10ms/11(GbISP_TFCellVoltHiFltLv2_flg)  "<GbISP_TFCellVoltHiFltLv2_flg>"
  Bus Selector6/1 -> BSD_250ms/1(GcSOC_DispSOC_pct)  "<GcSOC_DispSOC_pct>"
  BST_10ms/13(GeDCS_3513CurrFlt_enum) -> GeDCS_3513CurrFlt_enum/1
  BSM_250ms/4(GcDCS_3088MinTemp_C) -> GcDCS_3088MinTemp_C/1
  BCL_50ms/1(GcDCS_3072ChrgVoltReq_V) -> GcDCS_3072ChrgVoltReq_V/1
  BST_10ms/6(GeDCS_3512OutContOverTemp_enum) -> GeDCS_3512OutContOverTemp_enum/1
  BSM_250ms/11(GeDCS_3095OutContSt_enum) -> GeDCS_3095OutContSt_enum/1
  BCL_50ms/3(GeDCS_3074ChrgMode_enum) -> GeDCS_3074ChrgMode_enum/1
  BST_10ms/9(GeDCS_3512TempFlt_enum) -> GeDCS_3512TempFlt_enum/1
  BSM_250ms/7(GeDCS_3091SOCWarn_enum) -> GeDCS_3091SOCWarn_enum/1
  BST_10ms/1(GeDCS_3511ChrgrStop_enum) -> GeDCS_3511ChrgrStop_enum/1
  BSM_250ms/3(GcDCS_3087MaxTempIndex_numb) -> GcDCS_3087MaxTempIndex_numb/1
  BSM_250ms/9(GeDCS_3093TempWarn_enum) -> GeDCS_3093TempWarn_enum/1
  BSM_250ms/12(GeDCS_3096BMSChrgRdy_enum) -> GeDCS_3096BMSChrgRdy_enum/1
  BCS_250ms/1(GcDCS_3075ChrgVoltMea_V) -> GcDCS_3075ChrgVoltMea_V/1
  BCL_50ms/2(GcDCS_3073ChrgCurReq_A) -> GcDCS_3073ChrgCurReq_A/1
  BCS_250ms/6(GcDCS_3079TiRemain_min) -> GcDCS_3079TiRemain_min/1
  BST_10ms/3(GeDCS_3511ReachCellVolt_enum) -> GeDCS_3511ReachCellVolt_enum/1
  BST_10ms/10(GeDCS_3512HVRlyFlt_enum) -> GeDCS_3512HVRlyFlt_enum/1
  BSM_250ms/10(GeDCS_3094IsoState_enum) -> GeDCS_3094IsoState_enum/1
  BST_10ms/2(GeDCS_3511ReachSOC_enum) -> GeDCS_3511ReachSOC_enum/1
  BST_10ms/12(GeDCS_3512CC2VoltFlt_enum) -> GeDCS_3512CC2VoltFlt_enum/1
  BCS_250ms/3(GcDCS_3077MaxCellVolt_V) -> GcDCS_3077MaxCellVolt_V/1
  BST_10ms/7(GeDCS_3512BMSCompOverTemp_enum) -> GeDCS_3512BMSCompOverTemp_enum/1
  BST_10ms/8(GeDCS_3512ChrgContFlt_enum) -> GeDCS_3512ChrgContFlt_enum/1
  BSM_250ms/6(GeDCS_3090CellVoltWarn_enum) -> GeDCS_3090CellVoltWarn_enum/1
  BCS_250ms/5(GcDCS_3078SOC_pct) -> GcDCS_3078SOC_pct/1
  BSM_250ms/5(GcDCS_3089MinTempIndex_numb) -> GcDCS_3089MinTempIndex_numb/1
  BST_10ms/5(GeDCS_3512IsoFlt_enum) -> GeDCS_3512IsoFlt_enum/1
  BST_10ms/11(GeDCS_3512Other_enum) -> GeDCS_3512Other_enum/1
  BSM_250ms/8(GeDCS_3092CurWarn_enum) -> GeDCS_3092CurWarn_enum/1
  BSM_250ms/2(GcDCS_3086MaxTemp_C) -> GcDCS_3086MaxTemp_C/1
  BCS_250ms/4(GcDCS_3077MaxCellVoltGrp_numb) -> GcDCS_3077MaxCellVoltGrp_numb/1
  BCS_250ms/2(GcDCS_3076ChrgCurMea_A) -> GcDCS_3076ChrgCurMea_A/1
  BST_10ms/4(GeDCS_3511ReachPackVolt_enum) -> GeDCS_3511ReachPackVolt_enum/1
  BST_10ms/14(GeDCS_3513VoltFlt_enum) -> GeDCS_3513VoltFlt_enum/1
  BSM_250ms/1(GcDCS_3085MaxCellVoltIndex_numb) -> GcDCS_3085MaxCellVoltIndex_numb/1
  BEM_250ms/1(GeDCS_3901ToutCRM00_enum) -> GeDCS_3901ToutCRM00_enum/1
  BEM_250ms/8(GcDCS_BEMOther_numb) -> GcDCS_BEMOther_numb/1
  BEM_250ms/3(GeDCS_3903ToutCML_enum) -> GeDCS_3903ToutCML_enum/1
  BEM_250ms/5(GeDCS_3905ToutCCS_enum) -> GeDCS_3905ToutCCS_enum/1
  BEM_250ms/4(GeDCS_3904ToutCROAA_enum) -> GeDCS_3904ToutCROAA_enum/1
  BEM_250ms/7(GeDCS_3907ToutCSD_enum) -> GeDCS_3907ToutCSD_enum/1
  BEM_250ms/6(GeDCS_3906ToutCST_enum) -> GeDCS_3906ToutCST_enum/1
  BEM_250ms/2(GeDCS_3902ToutCRMAA_enum) -> GeDCS_3902ToutCRMAA_enum/1
  Bus Creator/1 -> Bus Selector9/1, Bus Selector1/1, Bus Selector8/1, Bus Selector2/1, Bus Selector3/1, Bus Selector4/1, Bus Selector5/1, Bus Selector6/1, Bus Selector7/1  "AllInput"
  DCS_BHM_250ms/1 -> BHM_250ms/Trigger
  DCS_BRM_250ms/1 -> BRM_250ms/Trigger
  DCS_BCL_50ms/1 -> BCL_50ms/Trigger
  DCS_BCS_250ms/1 -> BCS_250ms/Trigger
  DCS_BSM_250ms/1 -> BSM_250ms/Trigger
  DCS_BST_10ms/1 -> BST_10ms/Trigger
  DCS_BSD_250ms/1 -> BSD_250ms/Trigger
  DCS_BEM_250ms/1 -> BEM_250ms/Trigger
  DCS_BCP_500ms/1 -> BCP_500ms/Trigger
  DCS_BRO_250ms/1 -> BRO_250ms/Trigger
  BCP_500ms/1(GcDCS_2816MaxCellVoltPermit_V) -> GcDCS_2816MaxCellVoltPermit_V/1
  BCP_500ms/2(GcDCS_2817MaxCurPermit_A) -> GcDCS_2817MaxCurPermit_A/1
  BCP_500ms/3(GcDCS_2818RateEgy_Kwh) -> GcDCS_2818RateEgy_Kwh/1
  BCP_500ms/4(GcDCS_2819MaxVoltPermit_V) -> GcDCS_2819MaxVoltPermit_V/1
  BCP_500ms/5(GcDCS_2820MaxTempPermit_C) -> GcDCS_2820MaxTempPermit_C/1
  BCP_500ms/6(GcDCS_2821SOC_pct) -> GcDCS_2821SOC_pct/1
  BCP_500ms/7(GcDCS_2822PackVolt_V) -> GcDCS_2822PackVolt_V/1
  BRO_250ms/1(GcDCS_2829Da_numb) -> GcDCS_2829Da_numb/1
  Bus Selector8/2 -> BCP_500ms/2(GcHDP_PackVolt_V)  "<GcHDP_PackVolt_V>"
  Bus Selector8/1 -> BCP_500ms/1(GcSOC_DispSOC_pct)  "<GcSOC_DispSOC_pct>"
  Bus Selector9/1 -> BRO_250ms/1(GeCTC_CtrCtlState_enum)  "<GeCTC_CtrCtlState_enum>"
  Bus Selector7/8 -> BEM_250ms/8(GbDCC_CROTout_flg)  "<GbDCC_CROTout_flg>"
  Bus Selector5/12 -> BST_10ms/12(GbDCC_DCCrntUnctrolFlt_flg)  "<GbDCC_DCCrntUnctrolFlt_flg>"
  GbLDP_CC2STG_flg/1 -> BST_10ms/13(GbLDP_CC2STG_flg)
  GbLDP_CC2VoltRaty_flg/1 -> BST_10ms/14(GbLDP_CC2VoltRaty_flg)
  GcHDP_PackCrnt_A/1 -> Bus Creator/5  "GcHDP_PackCrnt_A"
  GcCDP_MaxCellVoltNumb_numb/1 -> Bus Creator/6  "GcCDP_MaxCellVoltNumb_numb"
  GcSOC_DispSOC_pct/1 -> Bus Creator/7  "GcSOC_DispSOC_pct"
  GcDCC_ChrgingTiRem_min/1 -> Bus Creator/8  "GcDCC_ChrgingTiRem_min"
  GcCDP_MaxCellTemp_C/1 -> Bus Creator/9  "GcCDP_MaxCellTemp_C"
  GcCDP_MaxCellTempNumb_numb/1 -> Bus Creator/10  "GcCDP_MaxCellTempNumb_numb"
  GcCDP_MinCellTemp_C/1 -> Bus Creator/11  "GcCDP_MinCellTemp_C"
  GcCDP_MinCellTempNumb_numb/1 -> Bus Creator/12  "GcCDP_MinCellTempNumb_numb"
  GbDCC_DCChrgFinish_flg/1 -> Bus Creator/13  "GbDCC_DCChrgFinish_flg"
  GeISO_ResFltLvl_enum/1 -> Bus Creator/14  "GeISO_ResFltLvl_enum"
  GeLDP_DCPlugTempState_enum/1 -> Bus Creator/15  "GeLDP_DCPlugTempState_enum"
  GbISP_TFCellTempHiFltLv2_flg/1 -> Bus Creator/16  "GbISP_TFCellTempHiFltLv2_flg"
  GbCTD_DCPosCloseFlt_flg/1 -> Bus Creator/17  "GbCTD_DCPosCloseFlt_flg"
  GbCTD_DCPosOpenFlt_flg/1 -> Bus Creator/18  "GbCTD_DCPosOpenFlt_flg"
  GeFTC_FltLevel_enum/1 -> Bus Creator/19  "GeFTC_FltLevel_enum"
  GeSOP_ChrgPwrState_enum/1 -> Bus Creator/20  "GeSOP_ChrgPwrState_enum"
  GbISP_TFCellVoltHiFltLv2_flg/1 -> Bus Creator/21  "GbISP_TFCellVoltHiFltLv2_flg"
  GcCDP_MinCellVolt_mV/1 -> Bus Creator/22  "GcCDP_MinCellVolt_mV"
  GcCDP_MaxCellVolt_mV/1 -> Bus Creator/23  "GcCDP_MaxCellVolt_mV"
  GbDCC_CRM00Tout_flg/1 -> Bus Creator/24  "GbDCC_CRM00Tout_flg"
  GbDCC_CRMAATout_flg/1 -> Bus Creator/25  "GbDCC_CRMAATout_flg"
  GbDCC_CMLTout_flg/1 -> Bus Creator/26  "GbDCC_CMLTout_flg"
  GbDCC_CROAATout_flg/1 -> Bus Creator/27  "GbDCC_CROAATout_flg"
  GbDCC_CCSTout_flg/1 -> Bus Creator/28  "GbDCC_CCSTout_flg"
  GbDCC_CSTTout_flg/1 -> Bus Creator/29  "GbDCC_CSTTout_flg"
  GbDCC_CSDTout_flg/1 -> Bus Creator/30  "GbDCC_CSDTout_flg"
  GbGDP_CSTRecOnce_flg/1 -> Bus Creator/31  "GbGDP_CSTRecOnce_flg"
  GcHDP_PackVolt_V/1 -> Bus Creator/32  "GcHDP_PackVolt_V"
  GeCTC_CtrCtlState_enum/1 -> Bus Creator/33  "GeCTC_CtrCtlState_enum"
  GbDCC_CROTout_flg/1 -> Bus Creator/34  "GbDCC_CROTout_flg"
  GbDCC_DCCrntUnctrolFlt_flg/1 -> Bus Creator/35  "GbDCC_DCCrntUnctrolFlt_flg"
  Bus Selector5/1 -> BST_10ms/1(GbDCC_BSTMsgCmd_flg)  "<GbDCC_BSTMsgCmd_flg>"
  GbDCC_BSTMsgCmd_flg/1 -> Bus Creator/1  "GbDCC_BSTMsgCmd_flg"
  GcADP_VinCode1_numb/1 -> BRM_250ms/2(GcADP_VinCode1_numb)  "GcADP_VinCode1_numb"
  GcADP_VinCode2_numb/1 -> BRM_250ms/3(GcADP_VinCode2_numb)  "GcADP_VinCode2_numb"
  GcADP_VinCode3_numb/1 -> BRM_250ms/4(GcADP_VinCode3_numb)  "GcADP_VinCode3_numb"
  GcADP_VinCode4_numb/1 -> BRM_250ms/5(GcADP_VinCode4_numb)  "GcADP_VinCode4_numb"
  GcADP_VinCode5_numb/1 -> BRM_250ms/6(GcADP_VinCode5_numb)  "GcADP_VinCode5_numb"
  GcADP_VinCode6_numb/1 -> BRM_250ms/7(GcADP_VinCode6_numb)  "GcADP_VinCode6_numb"
  GcADP_VinCode7_numb/1 -> BRM_250ms/8(GcADP_VinCode7_numb)  "GcADP_VinCode7_numb"
  GcADP_VinCodeNum_numb/1 -> BRM_250ms/9(GcADP_VinCodeNum_numb)  "GcADP_VinCodeNum_numb"
  GeCTC_CtrCtlConnMode_enum/1 -> Bus Creator/36  "GeCTC_CtrCtlConnMode_enum"
  Bus Selector9/2 -> BRO_250ms/2(GeCTC_CtrCtlConnMode_enum)  "<GeCTC_CtrCtlConnMode_enum>"
  Bus Selector2/3 -> BCL_50ms/3(GcHDP_PackVolt_V)  "<GcHDP_PackVolt_V>"

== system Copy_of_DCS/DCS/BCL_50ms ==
  GcDCC_DCChrgVoltRqst_V : Inport
  GcDCC_DCChrgCrntRqst_A : Inport  Port=2
  GcHDP_PackVolt_V : Inport  Port=3
  DCS_BCL_50ms : TriggerPort  TriggerType=function-call  VariantControl=(inherit)
  BCL_50ms_sys : Subsystem
  GcDCS_3072ChrgVoltReq_V : Outport
  GcDCS_3073ChrgCurReq_A : Outport  Port=2
  GeDCS_3074ChrgMode_enum : Outport  Port=3
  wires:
  GcDCC_DCChrgVoltRqst_V/1 -> BCL_50ms_sys/1(GcDCC_DCChrgVoltRqst_V)
  GcDCC_DCChrgCrntRqst_A/1 -> BCL_50ms_sys/2(GcDCC_DCChrgCrntRqst_A)
  BCL_50ms_sys/2(GcDCS_3073ChrgCurReq_A) -> GcDCS_3073ChrgCurReq_A/1
  BCL_50ms_sys/3(GeDCS_3074ChrgMode_enum) -> GeDCS_3074ChrgMode_enum/1
  BCL_50ms_sys/1(GcDCS_3072ChrgVoltReq_V) -> GcDCS_3072ChrgVoltReq_V/1
  GcHDP_PackVolt_V/1 -> BCL_50ms_sys/3(GcHDP_PackVolt_V)

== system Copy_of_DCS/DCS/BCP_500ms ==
  GcSOC_DispSOC_pct : Inport
  GcHDP_PackVolt_V : Inport  Port=2
  DCS_BCP_500ms : TriggerPort  TriggerType=function-call  VariantControl=(inherit)
  BCP_500ms_sys : Subsystem
  GcDCS_2816MaxCellVoltPermit_V : Outport
  GcDCS_2817MaxCurPermit_A : Outport  Port=2
  GcDCS_2818RateEgy_Kwh : Outport  Port=3
  GcDCS_2819MaxVoltPermit_V : Outport  Port=4
  GcDCS_2820MaxTempPermit_C : Outport  Port=5
  GcDCS_2821SOC_pct : Outport  Port=6
  GcDCS_2822PackVolt_V : Outport  Port=7
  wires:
  GcSOC_DispSOC_pct/1 -> BCP_500ms_sys/1(GcSOC_DispSOC_pct)
  GcHDP_PackVolt_V/1 -> BCP_500ms_sys/2(GcHDP_PackVolt_V)
  BCP_500ms_sys/1(GcDCS_2816MaxCellVoltPermit_V) -> GcDCS_2816MaxCellVoltPermit_V/1
  BCP_500ms_sys/2(GcDCS_2817MaxCurPermit_A) -> GcDCS_2817MaxCurPermit_A/1
  BCP_500ms_sys/3(GcDCS_2818RateEgy_Kwh) -> GcDCS_2818RateEgy_Kwh/1
  BCP_500ms_sys/4(GcDCS_2819MaxVoltPermit_V) -> GcDCS_2819MaxVoltPermit_V/1
  BCP_500ms_sys/5(GcDCS_2820MaxTempPermit_C) -> GcDCS_2820MaxTempPermit_C/1
  BCP_500ms_sys/6(GcDCS_2821SOC_pct) -> GcDCS_2821SOC_pct/1
  BCP_500ms_sys/7(GcDCS_2822PackVolt_V) -> GcDCS_2822PackVolt_V/1

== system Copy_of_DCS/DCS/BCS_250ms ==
  GcHDP_PackVolt_V : Inport
  GcHDP_PackCrnt_A : Inport  Port=2
  GcCDP_MaxCellVolt_mV : Inport  Port=3
  GcCDP_MaxCellVoltNumb_numb : Inport  Port=4
  GcSOC_DispSOC_pct : Inport  Port=5
  GcDCC_ChrgingTiRem_min : Inport  Port=6
  DCS_BCS_250ms : TriggerPort  TriggerType=function-call  VariantControl=(inherit)
  BCS_250ms_sys : Subsystem
  GcDCS_3075ChrgVoltMea_V : Outport
  GcDCS_3076ChrgCurMea_A : Outport  Port=2
  GcDCS_3077MaxCellVolt_V : Outport  Port=3
  GcDCS_3077MaxCellVoltGrp_numb : Outport  Port=4
  GcDCS_3078SOC_pct : Outport  Port=5
  GcDCS_3079TiRemain_min : Outport  Port=6
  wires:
  GcHDP_PackVolt_V/1 -> BCS_250ms_sys/1(GcHDP_PackVolt_V)
  GcHDP_PackCrnt_A/1 -> BCS_250ms_sys/2(GcHDP_PackCrnt_A)
  GcCDP_MaxCellVolt_mV/1 -> BCS_250ms_sys/3(GcCDP_MaxCellVolt_mV)
  GcSOC_DispSOC_pct/1 -> BCS_250ms_sys/5(GcSOC_DispSOC_pct)
  GcDCC_ChrgingTiRem_min/1 -> BCS_250ms_sys/6(GcDCC_ChrgingTiRem_min)
  GcCDP_MaxCellVoltNumb_numb/1 -> BCS_250ms_sys/4(GcCDP_MaxCellVoltNumb_numb)
  BCS_250ms_sys/1(GcDCS_3075ChrgVoltMea_V) -> GcDCS_3075ChrgVoltMea_V/1
  BCS_250ms_sys/2(GcDCS_3076ChrgCurMea_A) -> GcDCS_3076ChrgCurMea_A/1
  BCS_250ms_sys/6(GcDCS_3079TiRemain_min) -> GcDCS_3079TiRemain_min/1
  BCS_250ms_sys/5(GcDCS_3078SOC_pct) -> GcDCS_3078SOC_pct/1
  BCS_250ms_sys/4(GcDCS_3077MaxCellVoltGrp_numb) -> GcDCS_3077MaxCellVoltGrp_numb/1
  BCS_250ms_sys/3(GcDCS_3077MaxCellVolt_V) -> GcDCS_3077MaxCellVolt_V/1

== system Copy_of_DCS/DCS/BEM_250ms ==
  GbDCC_CRM00Tout_flg : Inport
  GbDCC_CRMAATout_flg : Inport  Port=2
  GbDCC_CMLTout_flg : Inport  Port=3
  GbDCC_CROAATout_flg : Inport  Port=4
  GbDCC_CCSTout_flg : Inport  Port=5
  GbDCC_CSTTout_flg : Inport  Port=6
  GbDCC_CSDTout_flg : Inport  Port=7
  GbDCC_CROTout_flg : Inport  Port=8
  DCS_BEM_250ms : TriggerPort  TriggerType=function-call  VariantControl=(inherit)
  BEM_250ms_sys : Subsystem
  GeDCS_3901ToutCRM00_enum : Outport
  GeDCS_3902ToutCRMAA_enum : Outport  Port=2
  GeDCS_3903ToutCML_enum : Outport  Port=3
  GeDCS_3904ToutCROAA_enum : Outport  Port=4
  GeDCS_3905ToutCCS_enum : Outport  Port=5
  GeDCS_3906ToutCST_enum : Outport  Port=6
  GeDCS_3907ToutCSD_enum : Outport  Port=7
  GcDCS_BEMOther_numb : Outport  Port=8
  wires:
  GbDCC_CRM00Tout_flg/1 -> BEM_250ms_sys/1(GbDCC_CRM00Tout_flg)
  GbDCC_CRMAATout_flg/1 -> BEM_250ms_sys/2(GbDCC_CRMAATout_flg)
  GbDCC_CMLTout_flg/1 -> BEM_250ms_sys/3(GbDCC_CMLTout_flg)
  GbDCC_CSDTout_flg/1 -> BEM_250ms_sys/7(GbDCC_CSDTout_flg)
  GbDCC_CROAATout_flg/1 -> BEM_250ms_sys/4(GbDCC_CROAATout_flg)
  GbDCC_CCSTout_flg/1 -> BEM_250ms_sys/5(GbDCC_CCSTout_flg)
  GbDCC_CSTTout_flg/1 -> BEM_250ms_sys/6(GbDCC_CSTTout_flg)
  BEM_250ms_sys/1(GeDCS_3901ToutCRM00_enum) -> GeDCS_3901ToutCRM00_enum/1
  BEM_250ms_sys/7(GeDCS_3907ToutCSD_enum) -> GeDCS_3907ToutCSD_enum/1
  BEM_250ms_sys/8(GcDCS_BEMOther_numb) -> GcDCS_BEMOther_numb/1
  BEM_250ms_sys/3(GeDCS_3903ToutCML_enum) -> GeDCS_3903ToutCML_enum/1
  BEM_250ms_sys/4(GeDCS_3904ToutCROAA_enum) -> GeDCS_3904ToutCROAA_enum/1
  BEM_250ms_sys/5(GeDCS_3905ToutCCS_enum) -> GeDCS_3905ToutCCS_enum/1
  BEM_250ms_sys/6(GeDCS_3906ToutCST_enum) -> GeDCS_3906ToutCST_enum/1
  BEM_250ms_sys/2(GeDCS_3902ToutCRMAA_enum) -> GeDCS_3902ToutCRMAA_enum/1
  GbDCC_CROTout_flg/1 -> BEM_250ms_sys/8(GbDCC_CROTout_flg)

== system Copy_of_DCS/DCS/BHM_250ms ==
  DCS_BHM_250ms : TriggerPort  TriggerType=function-call  VariantControl=(inherit)
  BHM_250ms_sys : Subsystem
  GcDCS_2601AlwMaxChrgVolt_V : Outport
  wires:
  BHM_250ms_sys/1(GcDCS_2601AlwMaxChrgVolt_V) -> GcDCS_2601AlwMaxChrgVolt_V/1

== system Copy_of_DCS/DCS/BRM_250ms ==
  GbDCC_DCChrgVerSta_flg : Inport
  GcADP_VinCode1_numb : Inport  Port=2
  GcADP_VinCode2_numb : Inport  Port=3
  GcADP_VinCode3_numb : Inport  Port=4
  GcADP_VinCode4_numb : Inport  Port=5
  GcADP_VinCode5_numb : Inport  Port=6
  GcADP_VinCode6_numb : Inport  Port=7
  GcADP_VinCode7_numb : Inport  Port=8
  GcADP_VinCodeNum_numb : Inport  Port=9
  DCS_BRM_250ms : TriggerPort  TriggerType=function-call  VariantControl=(inherit)
  BRM_250ms_sys : Subsystem
  GcDCS_2565ChrgVer_numb : Outport
  GeDCS_2566BattType_enum : Outport  Port=2
  GcDCS_2567BattCap_Ah : Outport  Port=3
  GcDCS_2568BattVolt_V : Outport  Port=4
  GaDCS_2569BattFctyName_numb : Outport  Port=5
  GcDCS_2570BattSer_numb : Outport  Port=6
  GcDCS_2571BattPrdctDay_D : Outport  Port=7
  GcDCS_2571BattPrdctMon_M : Outport  Port=8
  GcDCS_2571BattPrdctYr_Y : Outport  Port=9
  GcDCS_2572BattChrgCt_numb : Outport  Port=10
  GeDCS_2573BattPrpty_enum : Outport  Port=11
  GcDCS_2574Resv_numb : Outport  Port=12
  GaDCS_2575VIN_numb : Outport  Port=13
  GaDCS_2576SoftVer_numb : Outport  Port=14
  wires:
  BRM_250ms_sys/1(GcDCS_2565ChrgVer_numb) -> GcDCS_2565ChrgVer_numb/1
  BRM_250ms_sys/14(GaDCS_2576SoftVer_numb) -> GaDCS_2576SoftVer_numb/1
  BRM_250ms_sys/13(GaDCS_2575VIN_numb) -> GaDCS_2575VIN_numb/1
  BRM_250ms_sys/12(GcDCS_2574Resv_numb) -> GcDCS_2574Resv_numb/1
  BRM_250ms_sys/11(GeDCS_2573BattPrpty_enum) -> GeDCS_2573BattPrpty_enum/1
  BRM_250ms_sys/10(GcDCS_2572BattChrgCt_numb) -> GcDCS_2572BattChrgCt_numb/1
  BRM_250ms_sys/9(GcDCS_2571BattPrdctYr_Y) -> GcDCS_2571BattPrdctYr_Y/1
  BRM_250ms_sys/8(GcDCS_2571BattPrdctMon_M) -> GcDCS_2571BattPrdctMon_M/1
  BRM_250ms_sys/7(GcDCS_2571BattPrdctDay_D) -> GcDCS_2571BattPrdctDay_D/1
  BRM_250ms_sys/6(GcDCS_2570BattSer_numb) -> GcDCS_2570BattSer_numb/1
  BRM_250ms_sys/5(GaDCS_2569BattFctyName_numb) -> GaDCS_2569BattFctyName_numb/1
  BRM_250ms_sys/4(GcDCS_2568BattVolt_V) -> GcDCS_2568BattVolt_V/1
  BRM_250ms_sys/3(GcDCS_2567BattCap_Ah) -> GcDCS_2567BattCap_Ah/1
  BRM_250ms_sys/2(GeDCS_2566BattType_enum) -> GeDCS_2566BattType_enum/1
  GbDCC_DCChrgVerSta_flg/1 -> BRM_250ms_sys/1(GbDCC_DCChrgVerSta_flg)
  GcADP_VinCode1_numb/1 -> BRM_250ms_sys/2(GcADP_VinCode1_numb)
  GcADP_VinCode2_numb/1 -> BRM_250ms_sys/3(GcADP_VinCode2_numb)
  GcADP_VinCode3_numb/1 -> BRM_250ms_sys/4(GcADP_VinCode3_numb)
  GcADP_VinCode4_numb/1 -> BRM_250ms_sys/5(GcADP_VinCode4_numb)
  GcADP_VinCode5_numb/1 -> BRM_250ms_sys/6(GcADP_VinCode5_numb)
  GcADP_VinCode6_numb/1 -> BRM_250ms_sys/7(GcADP_VinCode6_numb)
  GcADP_VinCode7_numb/1 -> BRM_250ms_sys/8(GcADP_VinCode7_numb)
  GcADP_VinCodeNum_numb/1 -> BRM_250ms_sys/9(GcADP_VinCodeNum_numb)

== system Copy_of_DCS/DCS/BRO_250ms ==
  GeCTC_CtrCtlState_enum : Inport
  GeCTC_CtrCtlConnMode_enum : Inport  Port=2
  DCS_BRO_250ms : TriggerPort  TriggerType=function-call  VariantControl=(inherit)
  BRO_250ms_sys : Subsystem
  GcDCS_2829Da_numb : Outport
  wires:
  BRO_250ms_sys/1(GcDCS_2829Da_numb) -> GcDCS_2829Da_numb/1
  GeCTC_CtrCtlState_enum/1 -> BRO_250ms_sys/1(GeCTC_CtrCtlState_enum)
  GeCTC_CtrCtlConnMode_enum/1 -> BRO_250ms_sys/2(GeCTC_CtrCtlConnMode_enum)

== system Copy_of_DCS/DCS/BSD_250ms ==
  GcSOC_DispSOC_pct : Inport
  GcCDP_MinCellVolt_mV : Inport  Port=2
  GcCDP_MaxCellVolt_mV : Inport  Port=3
  GcCDP_MaxCellTemp_C : Inport  Port=4
  GcCDP_MinCellTemp_C : Inport  Port=5
  DCS_BSD_250ms : TriggerPort  TriggerType=function-call  VariantControl=(inherit)
  BSD_250ms_sys : Subsystem
  GcDCS_3601SOCFinal_pct : Outport
  GcDCS_3602MinCellVolt_V : Outport  Port=2
  GcDCS_3603MaxCellVolt_V : Outport  Port=3
  GcDCS_3604MinCellTemp_C : Outport  Port=4
  GcDCS_3605MaxCellTemp_C : Outport  Port=5
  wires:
  GcSOC_DispSOC_pct/1 -> BSD_250ms_sys/1(GcSOC_DispSOC_pct)
  GcCDP_MinCellVolt_mV/1 -> BSD_250ms_sys/2(GcCDP_MinCellVolt_mV)
  GcCDP_MaxCellVolt_mV/1 -> BSD_250ms_sys/3(GcCDP_MaxCellVolt_mV)
  GcCDP_MaxCellTemp_C/1 -> BSD_250ms_sys/4(GcCDP_MaxCellTemp_C)
  GcCDP_MinCellTemp_C/1 -> BSD_250ms_sys/5(GcCDP_MinCellTemp_C)
  BSD_250ms_sys/1(GcDCS_3601SOCFinal_pct) -> GcDCS_3601SOCFinal_pct/1
  BSD_250ms_sys/2(GcDCS_3602MinCellVolt_V) -> GcDCS_3602MinCellVolt_V/1
  BSD_250ms_sys/3(GcDCS_3603MaxCellVolt_V) -> GcDCS_3603MaxCellVolt_V/1
  BSD_250ms_sys/4(GcDCS_3604MinCellTemp_C) -> GcDCS_3604MinCellTemp_C/1
  BSD_250ms_sys/5(GcDCS_3605MaxCellTemp_C) -> GcDCS_3605MaxCellTemp_C/1

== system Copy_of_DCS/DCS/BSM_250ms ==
  GcCDP_MaxCellVoltNumb_numb : Inport
  GcCDP_MaxCellTemp_C : Inport  Port=2
  GcCDP_MaxCellTempNumb_numb : Inport  Port=3
  GcCDP_MinCellTemp_C : Inport  Port=4
  GcCDP_MinCellTempNumb_numb : Inport  Port=5
  DCS_BSM_250ms : TriggerPort  TriggerType=function-call  VariantControl=(inherit)
  BSM_250ms_sys : Subsystem
  GcDCS_3085MaxCellVoltIndex_numb : Outport
  GcDCS_3086MaxTemp_C : Outport  Port=2
  GcDCS_3087MaxTempIndex_numb : Outport  Port=3
  GcDCS_3088MinTemp_C : Outport  Port=4
  GcDCS_3089MinTempIndex_numb : Outport  Port=5
  GeDCS_3090CellVoltWarn_enum : Outport  Port=6
  GeDCS_3091SOCWarn_enum : Outport  Port=7
  GeDCS_3092CurWarn_enum : Outport  Port=8
  GeDCS_3093TempWarn_enum : Outport  Port=9
  GeDCS_3094IsoState_enum : Outport  Port=10
  GeDCS_3095OutContSt_enum : Outport  Port=11
  GeDCS_3096BMSChrgRdy_enum : Outport  Port=12
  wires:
  GcCDP_MaxCellVoltNumb_numb/1 -> BSM_250ms_sys/1(GcCDP_MaxCellVoltNumb_numb)
  GcCDP_MaxCellTemp_C/1 -> BSM_250ms_sys/2(GcCDP_MaxCellTemp_C)
  GcCDP_MaxCellTempNumb_numb/1 -> BSM_250ms_sys/3(GcCDP_MaxCellTempNumb_numb)
  GcCDP_MinCellTemp_C/1 -> BSM_250ms_sys/4(GcCDP_MinCellTemp_C)
  GcCDP_MinCellTempNumb_numb/1 -> BSM_250ms_sys/5(GcCDP_MinCellTempNumb_numb)
  BSM_250ms_sys/1(GcDCS_3085MaxCellVoltIndex_numb) -> GcDCS_3085MaxCellVoltIndex_numb/1
  BSM_250ms_sys/2(GcDCS_3086MaxTemp_C) -> GcDCS_3086MaxTemp_C/1
  BSM_250ms_sys/3(GcDCS_3087MaxTempIndex_numb) -> GcDCS_3087MaxTempIndex_numb/1
  BSM_250ms_sys/4(GcDCS_3088MinTemp_C) -> GcDCS_3088MinTemp_C/1
  BSM_250ms_sys/5(GcDCS_3089MinTempIndex_numb) -> GcDCS_3089MinTempIndex_numb/1
  BSM_250ms_sys/6(GeDCS_3090CellVoltWarn_enum) -> GeDCS_3090CellVoltWarn_enum/1
  BSM_250ms_sys/7(GeDCS_3091SOCWarn_enum) -> GeDCS_3091SOCWarn_enum/1
  BSM_250ms_sys/8(GeDCS_3092CurWarn_enum) -> GeDCS_3092CurWarn_enum/1
  BSM_250ms_sys/9(GeDCS_3093TempWarn_enum) -> GeDCS_3093TempWarn_enum/1
  BSM_250ms_sys/10(GeDCS_3094IsoState_enum) -> GeDCS_3094IsoState_enum/1
  BSM_250ms_sys/11(GeDCS_3095OutContSt_enum) -> GeDCS_3095OutContSt_enum/1
  BSM_250ms_sys/12(GeDCS_3096BMSChrgRdy_enum) -> GeDCS_3096BMSChrgRdy_enum/1

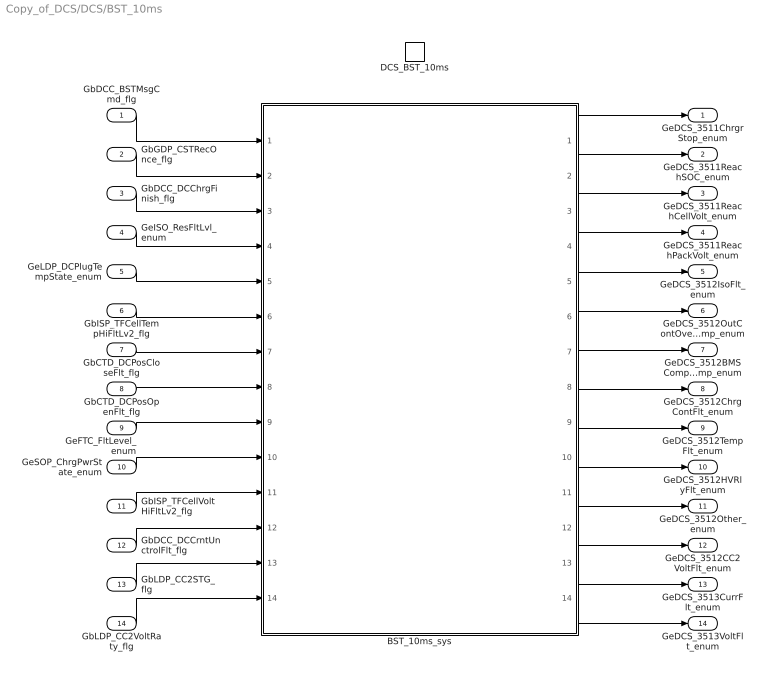
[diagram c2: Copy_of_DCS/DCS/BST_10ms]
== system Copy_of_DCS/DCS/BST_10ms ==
  GbDCC_BSTMsgCmd_flg : Inport
  GbGDP_CSTRecOnce_flg : Inport  Port=2
  GbDCC_DCChrgFinish_flg : Inport  Port=3
  GeISO_ResFltLvl_enum : Inport  Port=4
  GeLDP_DCPlugTempState_enum : Inport  Port=5
  GbISP_TFCellTempHiFltLv2_flg : Inport  Port=6
  GbCTD_DCPosCloseFlt_flg : Inport  Port=7
  GbCTD_DCPosOpenFlt_flg : Inport  Port=8
  GeFTC_FltLevel_enum : Inport  Port=9
  GeSOP_ChrgPwrState_enum : Inport  Port=10
  GbISP_TFCellVoltHiFltLv2_flg : Inport  Port=11
  GbDCC_DCCrntUnctrolFlt_flg : Inport  Port=12
  GbLDP_CC2STG_flg : Inport  Port=13
  GbLDP_CC2VoltRaty_flg : Inport  Port=14
  DCS_BST_10ms : TriggerPort  TriggerType=function-call  VariantControl=(inherit)
  BST_10ms_sys : Subsystem
  GeDCS_3511ChrgrStop_enum : Outport
  GeDCS_3511ReachSOC_enum : Outport  Port=2
  GeDCS_3511ReachCellVolt_enum : Outport  Port=3
  GeDCS_3511ReachPackVolt_enum : Outport  Port=4
  GeDCS_3512IsoFlt_enum : Outport  Port=5
  GeDCS_3512OutContOverTemp_enum : Outport  Port=6
  GeDCS_3512BMSCompOverTemp_enum : Outport  Port=7
  GeDCS_3512ChrgContFlt_enum : Outport  Port=8
  GeDCS_3512TempFlt_enum : Outport  Port=9
  GeDCS_3512HVRlyFlt_enum : Outport  Port=10
  GeDCS_3512Other_enum : Outport  Port=11
  GeDCS_3512CC2VoltFlt_enum : Outport  Port=12
  GeDCS_3513CurrFlt_enum : Outport  Port=13
  GeDCS_3513VoltFlt_enum : Outport  Port=14
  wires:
  GbISP_TFCellTempHiFltLv2_flg/1 -> BST_10ms_sys/6(GbISP_TFCellTempHiFltLv2_flg)
  GbCTD_DCPosOpenFlt_flg/1 -> BST_10ms_sys/8(GbCTD_DCPosOpenFlt_flg)
  GeLDP_DCPlugTempState_enum/1 -> BST_10ms_sys/5(GeLDP_DCPlugTempState_enum)
  GbDCC_DCChrgFinish_flg/1 -> BST_10ms_sys/3(GbDCC_DCChrgFinish_flg)
  GbCTD_DCPosCloseFlt_flg/1 -> BST_10ms_sys/7(GbCTD_DCPosCloseFlt_flg)
  GbDCC_BSTMsgCmd_flg/1 -> BST_10ms_sys/1(GbDCC_BSTMsgCmd_flg)
  GbGDP_CSTRecOnce_flg/1 -> BST_10ms_sys/2(GbGDP_CSTRecOnce_flg)
  GeISO_ResFltLvl_enum/1 -> BST_10ms_sys/4(GeISO_ResFltLvl_enum)
  GeFTC_FltLevel_enum/1 -> BST_10ms_sys/9(GeFTC_FltLevel_enum)
  GeSOP_ChrgPwrState_enum/1 -> BST_10ms_sys/10(GeSOP_ChrgPwrState_enum)
  GbISP_TFCellVoltHiFltLv2_flg/1 -> BST_10ms_sys/11(GbISP_TFCellVoltHiFltLv2_flg)
  BST_10ms_sys/1(GeDCS_3511ChrgrStop_enum) -> GeDCS_3511ChrgrStop_enum/1
  BST_10ms_sys/2(GeDCS_3511ReachSOC_enum) -> GeDCS_3511ReachSOC_enum/1
  BST_10ms_sys/3(GeDCS_3511ReachCellVolt_enum) -> GeDCS_3511ReachCellVolt_enum/1
  BST_10ms_sys/4(GeDCS_3511ReachPackVolt_enum) -> GeDCS_3511ReachPackVolt_enum/1
  BST_10ms_sys/5(GeDCS_3512IsoFlt_enum) -> GeDCS_3512IsoFlt_enum/1
  BST_10ms_sys/6(GeDCS_3512OutContOverTemp_enum) -> GeDCS_3512OutContOverTemp_enum/1
  BST_10ms_sys/7(GeDCS_3512BMSCompOverTemp_enum) -> GeDCS_3512BMSCompOverTemp_enum/1
  BST_10ms_sys/8(GeDCS_3512ChrgContFlt_enum) -> GeDCS_3512ChrgContFlt_enum/1
  BST_10ms_sys/9(GeDCS_3512TempFlt_enum) -> GeDCS_3512TempFlt_enum/1
  BST_10ms_sys/10(GeDCS_3512HVRlyFlt_enum) -> GeDCS_3512HVRlyFlt_enum/1
  BST_10ms_sys/11(GeDCS_3512Other_enum) -> GeDCS_3512Other_enum/1
  BST_10ms_sys/12(GeDCS_3512CC2VoltFlt_enum) -> GeDCS_3512CC2VoltFlt_enum/1
  BST_10ms_sys/13(GeDCS_3513CurrFlt_enum) -> GeDCS_3513CurrFlt_enum/1
  BST_10ms_sys/14(GeDCS_3513VoltFlt_enum) -> GeDCS_3513VoltFlt_enum/1
  GbDCC_DCCrntUnctrolFlt_flg/1 -> BST_10ms_sys/12(GbDCC_DCCrntUnctrolFlt_flg)
  GbLDP_CC2STG_flg/1 -> BST_10ms_sys/13(GbLDP_CC2STG_flg)
  GbLDP_CC2VoltRaty_flg/1 -> BST_10ms_sys/14(GbLDP_CC2VoltRaty_flg)
